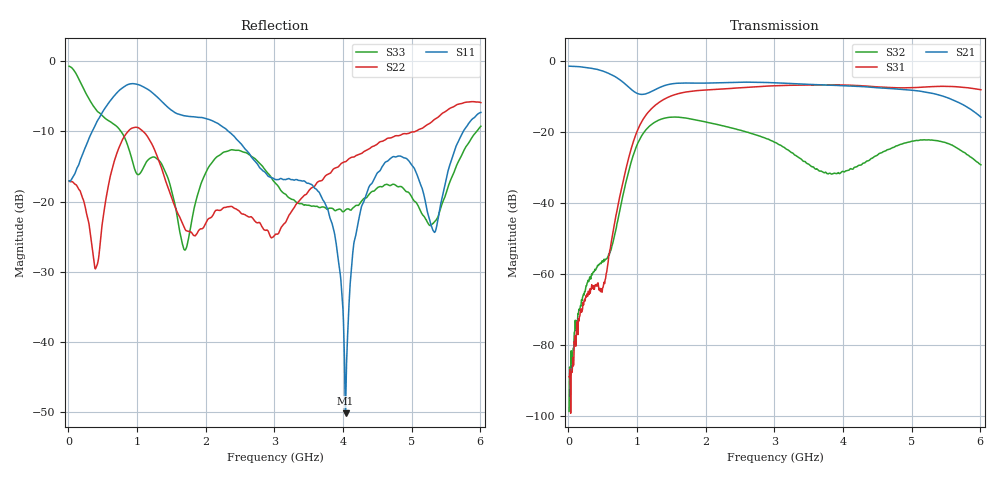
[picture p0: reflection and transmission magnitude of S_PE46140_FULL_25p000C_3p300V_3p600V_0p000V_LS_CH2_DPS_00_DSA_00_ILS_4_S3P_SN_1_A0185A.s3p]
! Device ID: PE46140_FULL
! File Path: z:\PE46140\MajorStates\25p000C\3p300\LS_CH2_DPS_00_DSA_00_ILS_4\PE46140_FULL_25p000C_3p300V_3p600V_0p000V_LS_CH2_DPS_00_DSA_00_ILS_4_S3P_SN_1_A0185A.s3p
! Serial: 1
! Lot: A0185A
! Temp: 25.000C
! VDD: 3.300
! VSS: 0.000
! Control_Hi: 3.600
! Control_Lo: 0.000
! Logic State: LS_CH2_DPS_00_DSA_00_ILS_4
! Port 1: RFIN
! Port 2: RFOUT1
! Port 3: RFOUT2
! ThroughPath:1-3
! IDD: 0.0003147296
! ISS: -2.092e-007
! Comment:
#  Hz  S  RI  R  50
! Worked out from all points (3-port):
!   801 points, 10 MHz to 6.01 GHz, reference 50 ohm
!   strongest paths, dB at 10 MHz, 1.51 GHz, 3.01 GHz, 4.51 GHz, 6.01 GHz:
!     S21: -1.5, -6.5, -6.2, -7.6, -15.9
!     S31: -88.9, -9.8, -7.0, -7.3, -8.1
!     S32: -98.7, -15.8, -23.0, -26.4, -29.3
!   lowest |S11| = -50.2 dB at 4.037 GHz (marker M1), VSWR 1.01, Z = 49.7 + j0.0889 ohm
!   |S11| at or under -10 dB: start of sweep to 346.2 MHz; 2.332 GHz to 5.753 GHz (3.421 GHz wide, 84.6 % of centre)
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1e7  0.1401 -0.0109  0.842 -0.0244  2.31e-05 3.22e-05
     0.8418 -0.0242  0.1399 -0.00674  1.88e-05 3.15e-05
     -3.56e-05 3.18e-06  -1.06e-05 4.83e-06  0.9175 -0.0871
3.55e8  -0.016 -0.3218  0.4592 -0.6282  -0.000571 -0.000266
        0.4593 -0.6262  -0.00913 -0.0426  -0.000184 0.00108
        -0.000587 -0.000339  -0.000153 0.00102  -0.4321 -0.2224
1.165e9  -0.5853 0.2238  -0.2048 -0.2879  -0.1879 -0.0281
         -0.2049 -0.2885  0.2133 -0.1871  -0.00305 0.1162
         -0.1882 -0.0284  -0.00316 0.1163  0.1669 0.1081
1.9825e9  -0.1842 0.3461  -0.418 0.2478  0.3836 -0.0567
          -0.4182 0.2478  0.0622 -0.0259  -0.1381 -0.0171
          0.3838 -0.0565  -0.1381 -0.0171  0.0443 0.1469
3.01e9  0.0194 0.1423  0.4091 0.2719  -0.3855 -0.2253
        0.4089 0.2729  -0.0577 -0.0014  0.0634 -0.0315
        -0.3856 -0.2256  0.0635 -0.0318  0.1281 -0.0462
3.76e9  0.0251 0.0886  0.2811 -0.3599  -0.2448 0.3884
        0.2818 -0.3596  0.0765 0.1342  -0.0159 0.0213
        -0.2449 0.3883  -0.0158 0.0211  0.0871 -0.017
4.0375e9  -0.00297 0.000895  0.0427 -0.4429  -0.00643 0.4561
          0.0433 -0.4432  0.1394 0.1325  0.0234 0.0152
          -0.00544 0.4556  0.0237 0.0151  0.0851 -0.0188
4.39e9  -0.1056 -0.0758  -0.2582 -0.3403  0.27 0.3455
        -0.2581 -0.3409  0.2177 0.098  0.014 -0.0377
        0.2703 0.3452  0.0142 -0.0377  0.1095 -0.0313
5.335e9  -0.0407 -0.0445  -0.108 0.3255  0.3187 -0.2964
         -0.1086 0.3257  0.383 -0.0377  0.0119 0.0746
         0.3191 -0.2958  0.0119 0.0749  0.0711 0.0101
6.01e9  -0.298 -0.3118  0.1535 0.0483  -0.1977 -0.3377
        0.1536 0.0485  0.2469 -0.4428  0.0287 -0.0186
        -0.1991 -0.3382  0.0289 -0.0187  0.317 0.1343
